| IBIS file created by T2B Version 16.0.0.01291   000
| Cadence Design Systems, Inc. 2011
| This Model is valid for  Temperature Range 0C<=Tc<=95C
| Valid for DDR4-2666/3200 operation
| Part Number   VDD/VDDQ/VPP   Package   Architecture
| SCB12Q8G800BF   1.2/1.2/2.5V   BGA96   32Meg x 16 x 4 x4
| SCB12Q8G160BF   1.2/1.2/2.5V   BGA78   64Meg x 16 x 4 x2
[IBIS ver] 5.1
[File name]  usssq8gxxbc.ibs
[File Rev]  1.0
[Date]   2024-10-20
[Source] Simulation of a silicon level SPICE model
[Notes]  IBIS Characteristics for I/O Buffer
   IBIS Model Revision History:
   Rev 1.0:   2024-10-20 - IBIS model file initial creation
[Disclaimer]  The IBIS models are for modeling purpose only and are
   subject to change without any notice. UniIC is not
   responsible for any problems the models may cause.
[Copyright] Copyright 2024 UniIC Semiconductors Corp. All rights reserved
|   Component SCB12Q8G800BF
[Component] SCB12Q8G800BF
[Manufacturer] UniIC Semiconductors Corp.
[Package]
| variable   typ   min   max
R_pkg   1.194E+00   4.721E-01   1.269E+00
L_pkg   2.286E-09   1.139E-09   2.957E-09
C_pkg   6.922E-13   3.827E-13   1.070E-12
[Pin]  signal_name   model_name   R_pin   L_pin   C_pin
A1   VDD   POWER
A2   VSSQ   GND
A3   TDQS_C   DQS   1.255E+00 2.287E-09 7.122E-13
A7   DML_N   DM   1.229E+00 2.267E-09 6.607E-13
A8   VSSQ   GND
A9   VSS   GND
B1   VPP   POWER
B2   VDDQ   POWER
B3   DQS_C   DQS   1.148E+00 2.621E-09 6.480E-13
B7   DQ1   DQ   1.269E+00 2.430E-09 6.790E-13
B8   VDDQ   POWER
B9   ZQ   NC   1.011E+00 2.372E-09 1.070E-12
C1   VDDQ   POWER
C2   DQ0   DQ   1.194E+00 2.286E-09 6.922E-13
C3   DQS_T   DQS   1.106E+00 2.497E-09 6.326E-13
C7   VDD   POWER
C8   VSS   GND
C9   VDDQ   POWER
D1   VSSQ   GND
D2   DQ4   DQ   1.211E+00 2.293E-09 6.836E-13
D3   DQ2   DQ   1.067E+00 2.180E-09 5.713E-13
D7   DQ3   DQ   1.129E+00 2.480E-09 5.863E-13
D8   DQ5   DQ   1.209E+00 2.215E-09 6.261E-13
D9   VSSQ   GND
E1   VSS   GND
E2   VDDQ   POWER
E3   DQ6   DQ   1.160E+00 2.135E-09 6.551E-13
E7   DQ7   DQ   1.120E+00 2.412E-09 5.608E-13
E8   VDDQ   POWER
E9   VSS   GND
F1   VDD   POWER
F2   NC   NC
F3   ODT   CA   6.040E-01 1.476E-09 5.579E-13
F7   CK_T   CK   1.002E+00 2.430E-09 5.673E-13
F8   CK_C   CK   1.090E+00 2.334E-09 6.490E-13
F9   VDD   POWER
G1   VSS   GND
G2   NC   NC
G3   CKE   CA   4.721E-01 1.139E-09 3.827E-13
G7   CS_N   CA   9.841E-01 2.211E-09 5.180E-13
G8   NC   NC
G9   TEN   TEN   1.155E+00 2.457E-09 7.762E-13
H1   VDD   POWER
H2   WE_N   CA   9.237E-01 2.324E-09 5.145E-13
H3   ACT_N   CA   9.496E-01 2.175E-09 4.810E-13
H7   CAS_N   CA   8.945E-01 2.432E-09 4.533E-13
H8   RAS_N   CA   1.085E+00 2.690E-09 5.823E-13
H9   VSS   GND
J1   VREFCA   POWER   9.683E-01 1.893E-09 7.138E-13
J2   BG0   CA   1.012E+00 2.282E-09 7.112E-13
J3   A10   CA   8.584E-01 2.214E-09 4.566E-13
J7   A12   CA   9.285E-01 2.706E-09 4.982E-13
J8   BG1   CA   1.061E+00 2.471E-09 7.249E-13
J9   VDD   POWER
K1   VSS   GND
K2   BA0   CA   1.023E+00 2.670E-09 5.599E-13
K3   A4   CA   8.382E-01 2.382E-09 4.362E-13
K7   A3   CA   1.070E+00 2.172E-09 6.251E-13
K8   BA1   CA   1.058E+00 2.514E-09 6.105E-13
K9   VSS   GND
L1   RESET_N   RST   1.002E+00 2.040E-09 6.940E-13
L2   A6   CA   9.088E-01 2.710E-09 5.430E-13
L3   A0   CA   8.538E-01 2.444E-09 4.578E-13
L7   A1   CA   1.049E+00 2.514E-09 5.929E-13
L8   A5   CA   9.532E-01 2.872E-09 5.141E-13
L9   ALERT_N   ALE   1.144E+00 2.386E-09 7.777E-13
M1   VDD   POWER
M2   A8   CA   9.806E-01 2.901E-09 5.735E-13
M3   A2   CA   9.092E-01 2.679E-09 5.101E-13
M7   A9   CA   9.017E-01 2.798E-09 4.755E-13
M8   A7   CA   9.783E-01 2.957E-09 5.169E-13
M9   VPP   POWER
N1   VSS   GND
N2   A11   CA   9.957E-01 2.902E-09 5.844E-13
N3   PAR   CA   1.085E+00 2.690E-09 5.823E-13
N7   NC   NC
N8   A13   CA   1.143E+00 2.607E-09 5.920E-13
N9   VDD   POWER
[Pin Mapping]  pulldown_ref   pullup_ref   gnd_clamp_ref   power_clamp_ref   ext_ref
A1   NC   VDD   NC   NC
A2   VSS   NC   NC   NC
A3   VSS   VDDQ   VSS   VDDQ
A7   VSS   VDDQ   VSS   VDDQ
A8   VSS   NC   NC   NC
A9   VSS   NC   NC   NC
B1   NC   VPP   NC   NC
B2   NC   VDDQ   NC   NC
B3   VSS   VDDQ   VSS   VDDQ
B7   VSS   VDDQ   VSS   VDDQ
B8   NC   VDDQ   NC   NC
B9   NC   NC   NC   NC
C1   NC   VDDQ   NC   NC
C2   VSS   VDDQ   VSS   VDDQ
C3   VSS   VDDQ   VSS   VDDQ
C7   NC   VDD   NC   NC
C8   VSS   NC   NC   NC
C9   NC   VDDQ   NC   NC
D1   VSS   NC   NC   NC
D2   VSS   VDDQ   VSS   VDDQ
D3   VSS   VDDQ   VSS   VDDQ
D7   VSS   VDDQ   VSS   VDDQ
D8   VSS   VDDQ   VSS   VDDQ
D9   VSS   NC   NC   NC
E1   VSS   NC   NC   NC
E2   NC   VDDQ   NC   NC
E3   VSS   VDDQ   VSS   VDDQ
E7   VSS   VDDQ   VSS   VDDQ
E8   NC   VDDQ   NC   NC
E9   VSS   NC   NC   NC
F1   NC   VDD   NC   NC
F2   NC   NC   NC   NC
F3   NC   NC   VSS   VDD
F7   NC   NC   VSS   VDD
F8   NC   NC   VSS   VDD
F9   NC   VDD   NC   NC
G1   VSS   NC   NC   NC
G2   NC   NC   NC   NC
G3   NC   NC   VSS   VDD
G7   NC   NC   VSS   VDD
G8   NC   NC   NC   NC
G9   NC   NC   VSS   VDD
H1   NC   VDD   NC   NC
H2   NC   NC   VSS   VDD
H3   NC   NC   VSS   VDD
H7   NC   NC   VSS   VDD
H8   NC   NC   VSS   VDD
H9   VSS   NC   NC   NC
J1   NC   VREFCA   NC   NC
J2   NC   NC   VSS   VDD
J3   NC   NC   VSS   VDD
J7   NC   NC   VSS   VDD
J8   NC   NC   VSS   VDD
J9   NC   VDD   NC   NC
K1   VSS   NC   NC   NC
K2   NC   NC   VSS   VDD
K3   NC   NC   VSS   VDD
K7   NC   NC   VSS   VDD
K8   NC   NC   VSS   VDD
K9   VSS   NC   NC   NC
L1   NC   NC   VSS   VDD
L2   NC   NC   VSS   VDD
L3   NC   NC   VSS   VDD
L7   NC   NC   VSS   VDD
L8   NC   NC   VSS   VDD
L9   VSS   VDD   VSS   VDD
M1   NC   VDD   NC   NC
M2   NC   NC   VSS   VDD
M3   NC   NC   VSS   VDD
M7   NC   NC   VSS   VDD
M8   NC   NC   VSS   VDD
M9   NC   VPP   NC   NC
N1   VSS   NC   NC   NC
N2   NC   NC   VSS   VDD
N3   NC   NC   VSS   VDD
N7   NC   NC   NC   NC
N8   NC   NC   VSS   VDD
N9   NC   VDD   NC   NC
[Diff pin]  inv_pin  vdiff   tdelay_typ   tdelay_min   tdelay_max
C3   B3   1.400E-01  NA   NA   0.000E+00
F7   F8   1.800E-01  NA   NA   0.000E+00
|   Component SCB12Q8G160BF
[Component] SCB12Q8G160BF
[Manufacturer] UniIC Semiconductors Corp.
[Package]
| variable   typ   min   max
R_pkg   1.079E+00   0.791E+00   1.522E+00
L_pkg   1.788E-09   1.466E-09   3.555E-09
C_pkg   0.576E-12   0.419E-12   0.877E-12
[Pin]  signal_name   model_name   R_pin   L_pin   C_pin
A1   VDDQ   POWER
A2   VSSQ   GND
A3   DQU0   DQ   1.079   1.788e-9  0.576e-12
A7   DQSU_C   DQS   1.0247   2.170e-9  0.531e-12
A8   VSSQ   GND
A9   VDDQ   POWER
B1   VPP   POWER
B2   VSS   GND
B3   VDD   POWER
B7   DQSU_T   DQS   1.064   3.101e-9	 0.565e-12
B8   DQU1   DQ   1.078   1.947e-9	 0.579e-12
B9   VDD   POWER
C1   VDDQ   POWER
C2   DQU4   DQ   1.026   1.664e-9	 0.551e-12
C3   DQU2   DQ   1.029   1.292e-9	 0.502e-12
C7   DQU3   DQ   0.990   1.888e-9	 0.491e-12
C8   DQU5   DQ   1.075   1.937e-9	 0.577e-12
C9   VSSQ   GND
D1   VDD   POWER
D2   VSSQ   GND
D3   DQU6   DQ   1.057   1.841e-9	 0.547e-12
D7   DQU7   DQ   1.018   1.815e-9	 0.559e-12
D8   VSSQ   GND
D9   VDDQ   POWER
E1   VSS   GND
E2   DMU_N   DM   1.075   1.726e-9	 0.565e-12
E3   VSSQ   GND
E7   DML_N   DM   0.896   1.514e-9	 0.501e-12
E8   VSSQ   GND
E9   VSS   GND
F1   VSSQ   GND
F2   VDDQ   POWER
F3   DQSL_C   DQS   0.887   1.675e-9	 0.499e-12
F7   DQL1   DQ   0.893   1.543e-9	 0.477e-12
F8   VDDQ   POWER
F9   ZQ   NC   0.791   1.729e-9	 0.767e-12
G1   VDDQ   POWER
G2   DQL0   DQ   0.927   1.636e-9	 0.514e-12
G3   DQSL_T   DQS   0.911   1.756e-9	 0.505e-12
G7   VDD   POWER
G8   VSS   GND
G9   VDDQ   POWER
H1   VSSQ   GND
H2   DQL4   DQ   0.946   1.689e-9	 0.516e-12
H3   DQL2   DQ   0.867   1.678e-9	 0.447e-12
H7   DQL3   DQ   0.898   1.484e-9	 0.503e-12
H8   DQL5   DQ   0.911   1.466e-9	 0.514e-12
H9   VSSQ   GND
J1   VDD   POWER
J2   VDDQ   POWER
J3   DQL6   DQ   0.858   1.646e-9	 0.440e-12
J7   DQL7   DQ   0.846   1.623e-9	 0.419e-12
J8   VDDQ   POWER
J9   VDD   POWER
K1   VSS   GND
K2   CKE   CA   1.005   1.915e-9	 0.545e-12
K3   ODT   CA   0.868   2.124e-9	 0.596e-12
K7   CK_T   CK   0.836   1.803e-9	 0.444e-12
K8   CK_C   CK   0.881   1.773e-9	 0.486e-12
K9   VSS   GND
L1   VDD   POWER
L2   WE_N   CA   1.371   2.569e-9	 0.604e-12
L3   ACT_N   CA   1.269   2.724e-9	 0.698e-12
L7   CS_N   CA   0.906   1.917e-9	 0.575e-12
L8   RAS_N   CA   1.380   2.822e-9	 0.700e-12
L9   VDD   POWER
M1   VREFCA   POWER   1.110   2.227e-9	 0.751e-12
M2   BG0   CA   1.296   2.966e-9	 0.580e-12
M3   A10   CA   1.213   2.839e-9	 0.635e-12
M7   A12   CA   1.254   2.897e-9	 0.575e-12
M8   CAS_N   CA   1.325   2.935e-9	 0.637e-12
M9   VSS   GND
N1   VSS   GND
N2   BA0   CA   1.395   3.082e-9	 0.650e-12
N3   A4   CA   1.359   2.578e-9	 0.569e-12
N7   A3   CA   1.236   2.832e-9	 0.588e-12
N8   BA1   CA   1.306   3.046e-9	 0.678e-12
N9   TEN   TEN   1.336   3.056e-9	 0.824e-12
P1   RESET_N   RST   1.419   2.502e-9	 0.829e-12
P2   A6   CA   1.342   3.342e-9	 0.624e-12
P3   A0   CA   1.279   3.179e-9	 0.685e-12
P7   A1   CA   1.251   3.124e-9	 0.699e-12
P8   A5   CA   1.347   3.299e-9	 0.645e-12
P9   ALERT_N   ALE   1.522   2.811e-9	 0.877e-12
R1   VDD   POWER
R2   A8   CA   1.401   3.555e-9	 0.680e-12
R3   A2   CA   1.323   3.428e-9	 0.607e-12
R7   A9   CA   1.266   3.207e-9	 0.620e-12
R8   A7   CA   1.352   3.392e-9	 0.673e-12
R9   VPP   POWER
T1   VSS   GND
T2   A11   CA   1.448   3.450e-9	 0.707e-12
T3   PAR   CA   1.455   2.922e-9	 0.720e-12
T7   NC   NC
T8   A13   CA   1.367   3.429e-9	 0.640e-12
T9   VDD   POWER
[Pin Mapping]  pulldown_ref   pullup_ref   gnd_clamp_ref   power_clamp_ref   ext_ref
A1	 NC	 VDDQ
A2	 VSSQ	 NC
A3	 VSS	 VDDQ	 VSS	 VDDQ
A7	 VSS	 VDDQ	 VSS	 VDDQ
A8	 VSSQ	 NC
A9	 NC	 VDDQ
B1	 NC	 VPP
B2	 VSS	 NC
B3	 NC	 VDD
B7	 VSS	 VDDQ	 VSS	 VDDQ
B8	 VSS	 VDDQ	 VSS	 VDDQ
B9	 NC	 VDD
C1	 NC	 VDDQ
C2	 VSS	 VDDQ	 VSS	 VDDQ
C3	 VSS	 VDDQ	 VSS	 VDDQ
C7	 VSS	 VDDQ	 VSS	 VDDQ
C8	 VSS	 VDDQ	 VSS	 VDDQ
C9	 VSSQ	 NC
D1	 NC	 VDD
D2	 VSSQ	 NC
D3	 VSS	 VDDQ	 VSS	 VDDQ
D7	 VSS	 VDDQ	 VSS	 VDDQ
D8	 VSSQ	 NC
D9	 NC	 VDDQ
E1	 VSS	 NC
E2	 VSS	 VDDQ	 VSS	 VDDQ
E3	 VSSQ	 NC
E7	 VSS	 VDDQ	 VSS	 VDDQ
E8	 VSSQ	 NC
E9	 VSS	 NC
F1	 VSSQ	 NC
F2	 NC	 VDDQ
F3	 VSS	 VDDQ	 VSS	 VDDQ
F7	 VSS	 VDDQ	 VSS	 VDDQ
F8	 NC	 VDDQ
F9	 NC	 NC
G1	 NC	 VDDQ
G2	 VSS	 VDDQ	 VSS	 VDDQ
G3	 VSS	 VDDQ	 VSS	 VDDQ
G7	 NC	 VDD
G8	 VSS	 NC
G9	 NC	 VDDQ
H1	 VSSQ	 NC
H2	 VSS	 VDDQ	 VSS	 VDDQ
H3	 VSS	 VDDQ	 VSS	 VDDQ
H7	 VSS	 VDDQ	 VSS	 VDDQ
H8	 VSS	 VDDQ	 VSS	 VDDQ
H9	 VSSQ	 NC
J1	 NC	 VDD
J2	 NC	 VDDQ
J3	 VSS	 VDDQ	 VSS	 VDDQ
J7	 VSS	 VDDQ	 VSS	 VDDQ
J8	 NC	 VDDQ
J9	 NC	 VDD
K1	 VSS	 NC
K2	 NC	 NC	 VSS	 VDD
K3	 NC	 NC	 VSS	 VDD
K7	 NC	 NC	 VSS	 VDD
K8	 NC	 NC	 VSS	 VDD
K9	 VSS	 NC
L1	 NC	 VDD
L2	 NC	 NC	 VSS	 VDD
L3	 NC	 NC	 VSS	 VDD
L7	 NC	 NC	 VSS	 VDD
L8	 NC	 NC	 VSS	 VDD
L9	 NC	 VDD
M1	 NC	 VREFCA
M2	 NC	 NC	 VSS	 VDD
M3	 NC	 NC	 VSS	 VDD
M7	 NC	 NC	 VSS	 VDD
M8	 NC	 NC	 VSS	 VDD
M9	 VSS	 NC
N1	 VSS	 NC
N2	 NC	 NC	 VSS	 VDD
N3	 NC	 NC	 VSS	 VDD
N7	 NC	 NC	 VSS	 VDD
N8	 NC	 NC	 VSS	 VDD
N9	 NC	 NC	 VSS	 VDD
P1	 NC	 NC	 VSS	 VDD
P2	 NC	 NC	 VSS	 VDD
P3	 NC	 NC	 VSS	 VDD
P7	 NC	 NC	 VSS	 VDD
P8	 NC	 NC	 VSS	 VDD
P9	 VSS	 VDD	 VSS	 VDD
R1	 NC	 VDD
R2	 NC	 NC	 VSS	 VDD
R3	 NC	 NC	 VSS	 VDD
R7	 NC	 NC	 VSS	 VDD
R8	 NC	 NC	 VSS	 VDD
R9	 NC	 VPP
T1	 VSS	 NC
T2	 NC	 NC	 VSS	 VDD
T3	 NC	 NC	 VSS	 VDD
T7	 NC	 NC
T8	 NC	 NC	 VSS	 VDD
T9	 NC	 VDD
[Diff pin]  inv_pin  vdiff   tdelay_typ   tdelay_min   tdelay_max
B7	 A7	 1.400E-01	 NA	 NA	 0.000E+00
G3	 F3	 1.400E-01	 NA	 NA	 0.000E+00
K7	 K8	 1.800E-01	 NA	 NA	 0.000E+00
[Model Selector] DQ
DQ_34 34 Ohm Data I/O with no ODT
DQ_48 48 Ohm Data I/O with no ODT
DQ_ODT_34 Data Input with 34 Ohm ODT
DQ_ODT_40 Data Input with 40 Ohm ODT
DQ_ODT_48 Data Input with 48 Ohm ODT
DQ_ODT_60 Data Input with 60 Ohm ODT
DQ_ODT_80 Data Input with 80 Ohm ODT
DQ_ODT_120 Data Input with 120 Ohm ODT
DQ_ODT_240 Data Input with 240 Ohm ODT
DQ_ODT_OFF Data Input with no ODT
[Model Selector] DQS
DQS_34 34 Ohm Data Strobe I/O with no ODT
DQS_48 48 Ohm Data Strobe I/O with no ODT
DQS_ODT_34 Data Strobe Input with 34 Ohm ODT
DQS_ODT_40 Data Strobe Input with 40 Ohm ODT
DQS_ODT_48 Data Strobe Input with 48 Ohm ODT
DQS_ODT_60 Data Strobe Input with 60 Ohm ODT
DQS_ODT_80 Data Strobe Input with 80 Ohm ODT
DQS_ODT_120 Data Strobe Input with 120 Ohm ODT
DQS_ODT_240 Data Strobe Input with 240 Ohm ODT
DQS_ODT_OFF Data Strobe Input with no ODT
[Model Selector] DM
DQ_34 34 Ohm Data I/O with no ODT
DQ_48 48 Ohm Data I/O with no ODT
DQ_ODT_34 Data Input with 34 Ohm ODT
DQ_ODT_40 Data Input with 40 Ohm ODT
DQ_ODT_48 Data Input with 48 Ohm ODT
DQ_ODT_60 Data Input with 60 Ohm ODT
DQ_ODT_80 Data Input with 80 Ohm ODT
DQ_ODT_120 Data Input with 120 Ohm ODT
DQ_ODT_240 Data Input with 240 Ohm ODT
DQ_ODT_OFF Data Input with no ODT
[Model Selector] ALE
ALE_DRV ALERT_N Data I/O with no ODT
ALE_RCV Data Input with no ODT
| Models and submodels in the file (26): DQ_34 (I/O), DQ_48 (I/O), DQ_ODT_34 (Input), DQ_ODT_40 (Input), DQ_ODT_48 (Input), DQ_ODT_60 (Input), DQ_ODT_80 (Input), DQ_ODT_120 (Input), DQ_ODT_240 (Input), DQ_ODT_OFF (Input), DQS_34 (I/O), DQS_48 (I/O), DQS_ODT_34 (Input), DQS_ODT_40 (Input), DQS_ODT_48 (Input), DQS_ODT_60 (Input), DQS_ODT_80 (Input), DQS_ODT_120 (Input), DQS_ODT_240 (Input), DQS_ODT_OFF (Input), ALE_DRV (Open_sink), ALE_RCV (Input), CA (Input), CK (Input), RST (Input), TEN (Input)
